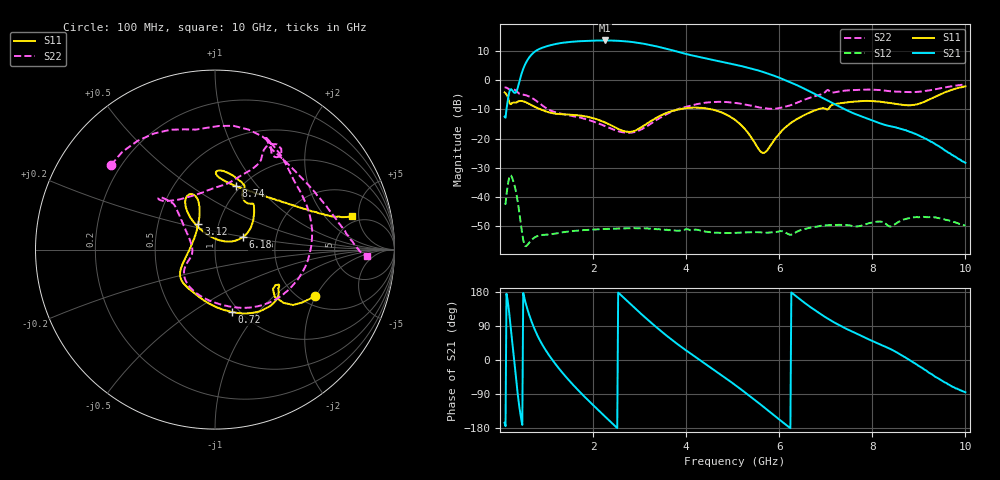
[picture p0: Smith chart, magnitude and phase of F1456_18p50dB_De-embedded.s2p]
! Integrated Device Technology
! Corporate Headquarters
! 6024 Silver Creek Valley Road
! San Jose, CA 95138  USA
! Phone:  1-408-284-8200
! Toll Free:  1-800-223-1366
! Webpage:  http://www.idt.com/
! Timing and RF Division
! 515 Groton Road, Suite 102
! Westford, MA 01886-6024
! Device:  F1456
! Description: 6-bit 0.5 dB Transmit Variable Gain Amplifier
! Frequency:  2100.0 -  2950.00 MHz
! Package:  6x6 mm Thin QFN Plastic Package: 28 pin
! State:  37
! Atten State:  18.5 dB
! Voltage:  +5.00 Volts
! Current:  216.966 mA
! Data:  The device was measured on a the F1455 evaluation board which has
!  individual transmission lines to the RF pins.  Data was collected
!  using a calibrated network analyzer.  The evaluation board was
!  de-embedded using a TRL calibration technique.
!  The reference plane is the edge of the package pin.
!  Pin  1 = CSb
!  Pin  2 = DATA
!  Pin  3 = CLK
!  Pin  4 = RSET
!  Pin  5 = GND
!  Pin  6 = RFIN  = Port 1
!  Pin  7 = GND
!  Pin  8 = NC
!  Pin  9 = NC
!  Pin 10 = NC
!  Pin 11 = NC
!  Pin 12 = NC
!  Pin 13 = NC
!  Pin 14 = /STBY
!  Pin 15 = GND
!  Pin 16 = RFOUT  = Port 2
!  Pin 17 = GND
!  Pin 18 = NC
!  Pin 19 = NC
!  Pin 20 = NC
!  Pin 21 = GND
!  Pin 22 = NC
!  Pin 23 = GND
!  Pin 24 = NC
!  Pin 25 = NC
!  Pin 26 = NC
!  Pin 27 = GND
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# GHz S dB R 50
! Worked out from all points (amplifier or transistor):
!   496 points, 100 MHz to 10 GHz, reference 50 ohm
!   highest |S21| = 13.6 dB at 2.26 GHz (marker M1)
!   |S21| within 3 dB of that: 833.9 MHz to 3.615 GHz (2.781 GHz wide, 125 % of centre)
!   unconditionally stable (mu >= 1): start of sweep to end of sweep
!   at 1.74 GHz: K = 35.34, MAG = 13.8 dB, |S12| = -51.3 dB
!   at 5.06 GHz: K = 88.06, MAG = 6.3 dB, |S12| = -52.2 dB
!   at 10 GHz: K = 432.48, MAG = -18.7 dB, |S12| = -49.7 dB
!   S11 on the Smith chart (normalised r, x): 100 MHz: 2.36, -1.99; 720 MHz: 0.92, -0.74; 3.12 GHz: 0.80, +0.24; 6.18 GHz: 1.35, +0.19; 8.74 GHz: 0.95, +0.78; 10 GHz: 4.19, +4.08
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0.1  -4.19 -25.0  -12.45 -165.6  -42.32 48.6  -2.54 140.8
0.3  -7.66 -30.9  -4.19 7.1  -35.23 -133.6  -3.17 74.5
0.42  -7.11 -37.8  -0.27 -127.0  -45.72 141.7  -4.64 41.7
0.56  -7.59 -56.6  6.01 146.8  -56.73 151.1  -5.15 11.6
0.72  -8.85 -74.8  9.37 88.5  -54.03 138.9  -6.41 -24.2
0.96  -10.54 -98.5  11.36 30.3  -52.86 95.5  -9.22 -69.0
1.18  -11.42 -115.4  12.31 -8.7  -52.46 71.8  -10.91 -97.0
1.48  -11.76 -131.6  13.03 -53.2  -51.69 48.0  -11.99 -123.9
1.76  -12.18 -142.1  13.35 -89.7  -51.30 30.6  -12.94 -139.7
2  -12.97 -149.0  13.51 -118.8  -51.07 17.8  -14.10 -148.7
2.26  -14.46 -158.4  13.57 -149.5  -50.85 5.1  -15.72 -156.5
2.64  -17.33 173.7  13.35 166.4  -50.70 -12.6  -17.82 -171.5
3.12  -15.28 122.5  12.36 112.2  -50.68 -36.4  -16.13 156.7
3.4  -12.52 111.3  11.42 82.4  -50.93 -49.1  -13.28 142.7
4.08  -9.44 113.2  8.64 18.5  -51.25 -79.5  -8.78 132.9
5.06  -13.69 127.8  5.28 -66.7  -52.16 -125.7  -7.77 137.8
5.66  -24.87 71.2  2.77 -123.4  -52.10 -161.2  -9.55 120.0
6.18  -15.47 23.9  -0.38 -174.3  -52.46 164.8  -8.82 82.9
6.7  -10.77 41.5  -4.19 137.0  -50.31 143.2  -5.81 64.3
8.36  -7.75 88.1  -15.64 31.0  -49.96 70.1  -3.75 62.4
8.74  -8.54 72.0  -17.28 4.5  -47.37 65.7  -4.07 49.1
10  -2.11 13.8  -28.25 -85.1  -49.67 -22.8  -1.46 -2.6
